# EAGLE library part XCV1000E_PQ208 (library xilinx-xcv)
xcv1000e_pq208 edit this description Auto generated by make-symbol-device-package-bsdl.ulp Rev. 26 Source: xcv1000e_pq208.bsd
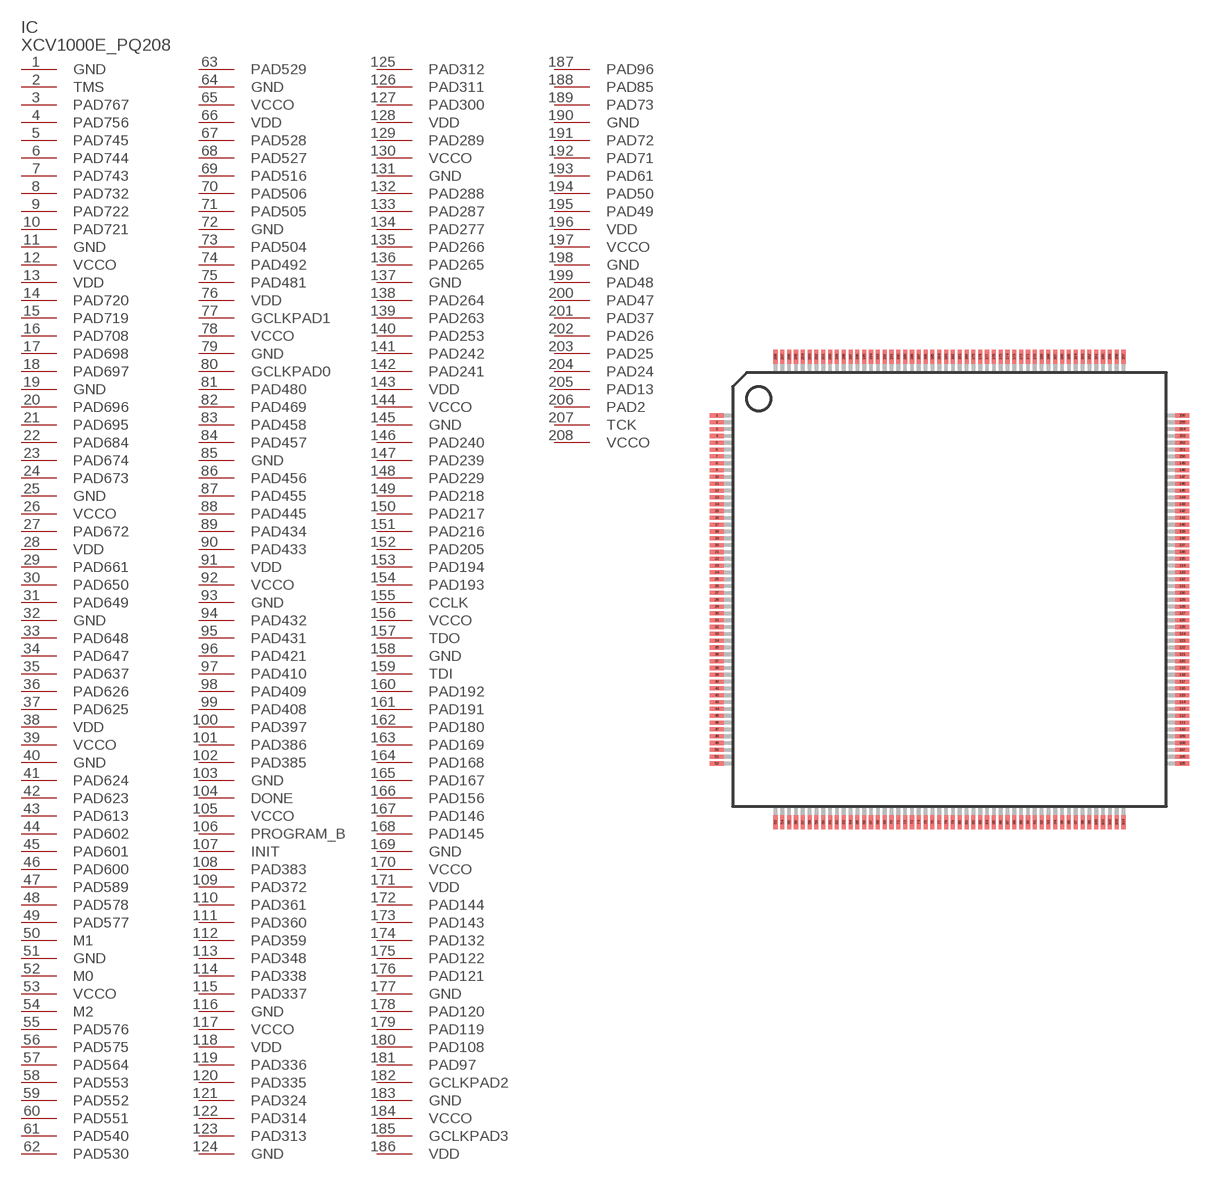
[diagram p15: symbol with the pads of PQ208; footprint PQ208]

Designator prefix IC

## XCV1000E_PQ208 (OC_FARNELL: unknown; OC_NEWARK: unknown)  [PQ208]
1  GND  pwr
2  TMS  in
3  PAD767
4  PAD756
5  PAD745
6  PAD744
7  PAD743
8  PAD732
9  PAD722
10  PAD721
11  GND  pwr
12  VCCO  pwr
13  VDD  pwr
14  PAD720
15  PAD719
16  PAD708
17  PAD698
18  PAD697
19  GND  pwr
20  PAD696
21  PAD695
22  PAD684
23  PAD674
24  PAD673
25  GND  pwr
26  VCCO  pwr
27  PAD672
28  VDD  pwr
29  PAD661
30  PAD650
31  PAD649
32  GND  pwr
33  PAD648
34  PAD647
35  PAD637
36  PAD626
37  PAD625
38  VDD  pwr
39  VCCO  pwr
40  GND  pwr
41  PAD624
42  PAD623
43  PAD613
44  PAD602
45  PAD601
46  PAD600
47  PAD589
48  PAD578
49  PAD577
50  M1  in
51  GND  pwr
52  M0  in
53  VCCO  pwr
54  M2  in
55  PAD576
56  PAD575
57  PAD564
58  PAD553
59  PAD552
60  PAD551
61  PAD540
62  PAD530
63  PAD529
64  GND  pwr
65  VCCO  pwr
66  VDD  pwr
67  PAD528
68  PAD527
69  PAD516
70  PAD506
71  PAD505
72  GND  pwr
73  PAD504
74  PAD492
75  PAD481
76  VDD  pwr
77  GCLKPAD1  in
78  VCCO  pwr
79  GND  pwr
80  GCLKPAD0  in
81  PAD480
82  PAD469
83  PAD458
84  PAD457
85  GND  pwr
86  PAD456
87  PAD455
88  PAD445
89  PAD434
90  PAD433
91  VDD  pwr
92  VCCO  pwr
93  GND  pwr
94  PAD432
95  PAD431
96  PAD421
97  PAD410
98  PAD409
99  PAD408
100  PAD397
101  PAD386
102  PAD385
103  GND  pwr
104  DONE
105  VCCO  pwr
106  PROGRAM_B  in
107  INIT
108  PAD383
109  PAD372
110  PAD361
111  PAD360
112  PAD359
113  PAD348
114  PAD338
115  PAD337
116  GND  pwr
117  VCCO  pwr
118  VDD  pwr
119  PAD336
120  PAD335
121  PAD324
122  PAD314
123  PAD313
124  GND  pwr
125  PAD312
126  PAD311
127  PAD300
128  VDD  pwr
129  PAD289
130  VCCO  pwr
131  GND  pwr
132  PAD288
133  PAD287
134  PAD277
135  PAD266
136  PAD265
137  GND  pwr
138  PAD264
139  PAD263
140  PAD253
141  PAD242
142  PAD241
143  VDD  pwr
144  VCCO  pwr
145  GND  pwr
146  PAD240
147  PAD239
148  PAD229
149  PAD218
150  PAD217
151  PAD216
152  PAD205
153  PAD194
154  PAD193
155  CCLK
156  VCCO  pwr
157  TDO  out
158  GND  pwr
159  TDI  in
160  PAD192
161  PAD191
162  PAD180
163  PAD169
164  PAD168
165  PAD167
166  PAD156
167  PAD146
168  PAD145
169  GND  pwr
170  VCCO  pwr
171  VDD  pwr
172  PAD144
173  PAD143
174  PAD132
175  PAD122
176  PAD121
177  GND  pwr
178  PAD120
179  PAD119
180  PAD108
181  PAD97
182  GCLKPAD2  in
183  GND  pwr
184  VCCO  pwr
185  GCLKPAD3  in
186  VDD  pwr
187  PAD96
188  PAD85
189  PAD73
190  GND  pwr
191  PAD72
192  PAD71
193  PAD61
194  PAD50
195  PAD49
196  VDD  pwr
197  VCCO  pwr
198  GND  pwr
199  PAD48
200  PAD47
201  PAD37
202  PAD26
203  PAD25
204  PAD24
205  PAD13
206  PAD2
207  TCK  in
208  VCCO  pwr

## Footprint PQ208 (pad centres in mm)
PQ208 Auto generated by make-symbol-device-package-bsdl.ulp Rev. 26
smd 1 x 0.3: 1 -17.05,12.75; 2 -17.05,12.25; 3 -17.05,11.75; 4 -17.05,11.25; 5 -17.05,10.75; 6 -17.05,10.25; 7 -17.05,9.75; 8 -17.05,9.25; 9 -17.05,8.75; 10 -17.05,8.25; 11 -17.05,7.75; 12 -17.05,7.25; 13 -17.05,6.75; 14 -17.05,6.25; 15 -17.05,5.75; 16 -17.05,5.25; 17 -17.05,4.75; 18 -17.05,4.25; 19 -17.05,3.75; 20 -17.05,3.25; 21 -17.05,2.75; 22 -17.05,2.25; 23 -17.05,1.75; 24 -17.05,1.25; 25 -17.05,0.75; 26 -17.05,0.25; 27 -17.05,-0.25; 28 -17.05,-0.75; 29 -17.05,-1.25; 30 -17.05,-1.75; 31 -17.05,-2.25; 32 -17.05,-2.75; 33 -17.05,-3.25; 34 -17.05,-3.75; 35 -17.05,-4.25; 36 -17.05,-4.75; 37 -17.05,-5.25; 38 -17.05,-5.75; 39 -17.05,-6.25; 40 -17.05,-6.75; 41 -17.05,-7.25; 42 -17.05,-7.75; 43 -17.05,-8.25; 44 -17.05,-8.75; 45 -17.05,-9.25; 46 -17.05,-9.75; 47 -17.05,-10.25; 48 -17.05,-10.75; 49 -17.05,-11.25; 50 -17.05,-11.75; 51 -17.05,-12.25; 52 -17.05,-12.75; 105 17.05,-12.75; 106 17.05,-12.25; 107 17.05,-11.75; 108 17.05,-11.25; 109 17.05,-10.75; 110 17.05,-10.25; 111 17.05,-9.75; 112 17.05,-9.25; 113 17.05,-8.75; 114 17.05,-8.25; 115 17.05,-7.75; 116 17.05,-7.25; 117 17.05,-6.75; 118 17.05,-6.25; 119 17.05,-5.75; 120 17.05,-5.25; 121 17.05,-4.75; 122 17.05,-4.25; 123 17.05,-3.75; 124 17.05,-3.25; 125 17.05,-2.75; 126 17.05,-2.25; 127 17.05,-1.75; 128 17.05,-1.25; 129 17.05,-0.75; 130 17.05,-0.25; 131 17.05,0.25; 132 17.05,0.75; 133 17.05,1.25; 134 17.05,1.75; 135 17.05,2.25; 136 17.05,2.75; 137 17.05,3.25; 138 17.05,3.75; 139 17.05,4.25; 140 17.05,4.75; 141 17.05,5.25; 142 17.05,5.75; 143 17.05,6.25; 144 17.05,6.75; 145 17.05,7.25; 146 17.05,7.75; 147 17.05,8.25; 148 17.05,8.75; 149 17.05,9.25; 150 17.05,9.75; 151 17.05,10.25; 152 17.05,10.75; 153 17.05,11.25; 154 17.05,11.75; 155 17.05,12.25; 156 17.05,12.75
smd 0.3 x 1: 53 -12.75,-17.05; 54 -12.25,-17.05; 55 -11.75,-17.05; 56 -11.25,-17.05; 57 -10.75,-17.05; 58 -10.25,-17.05; 59 -9.75,-17.05; 60 -9.25,-17.05; 61 -8.75,-17.05; 62 -8.25,-17.05; 63 -7.75,-17.05; 64 -7.25,-17.05; 65 -6.75,-17.05; 66 -6.25,-17.05; 67 -5.75,-17.05; 68 -5.25,-17.05; 69 -4.75,-17.05; 70 -4.25,-17.05; 71 -3.75,-17.05; 72 -3.25,-17.05; 73 -2.75,-17.05; 74 -2.25,-17.05; 75 -1.75,-17.05; 76 -1.25,-17.05; 77 -0.75,-17.05; 78 -0.25,-17.05; 79 0.25,-17.05; 80 0.75,-17.05; 81 1.25,-17.05; 82 1.75,-17.05; 83 2.25,-17.05; 84 2.75,-17.05; 85 3.25,-17.05; 86 3.75,-17.05; 87 4.25,-17.05; 88 4.75,-17.05; 89 5.25,-17.05; 90 5.75,-17.05; 91 6.25,-17.05; 92 6.75,-17.05; 93 7.25,-17.05; 94 7.75,-17.05; 95 8.25,-17.05; 96 8.75,-17.05; 97 9.25,-17.05; 98 9.75,-17.05; 99 10.25,-17.05; 100 10.75,-17.05; 101 11.25,-17.05; 102 11.75,-17.05; 103 12.25,-17.05; 104 12.75,-17.05; 157 12.75,17.05; 158 12.25,17.05; 159 11.75,17.05; 160 11.25,17.05; 161 10.75,17.05; 162 10.25,17.05; 163 9.75,17.05; 164 9.25,17.05; 165 8.75,17.05; 166 8.25,17.05; 167 7.75,17.05; 168 7.25,17.05; 169 6.75,17.05; 170 6.25,17.05; 171 5.75,17.05; 172 5.25,17.05; 173 4.75,17.05; 174 4.25,17.05; 175 3.75,17.05; 176 3.25,17.05; 177 2.75,17.05; 178 2.25,17.05; 179 1.75,17.05; 180 1.25,17.05; 181 0.75,17.05; 182 0.25,17.05; 183 -0.25,17.05; 184 -0.75,17.05; 185 -1.25,17.05; 186 -1.75,17.05; 187 -2.25,17.05; 188 -2.75,17.05; 189 -3.25,17.05; 190 -3.75,17.05; 191 -4.25,17.05; 192 -4.75,17.05; 193 -5.25,17.05; 194 -5.75,17.05; 195 -6.25,17.05; 196 -6.75,17.05; 197 -7.25,17.05; 198 -7.75,17.05; 199 -8.25,17.05; 200 -8.75,17.05; 201 -9.25,17.05; 202 -9.75,17.05; 203 -10.25,17.05; 204 -10.75,17.05; 205 -11.25,17.05; 206 -11.75,17.05; 207 -12.25,17.05; 208 -12.75,17.05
